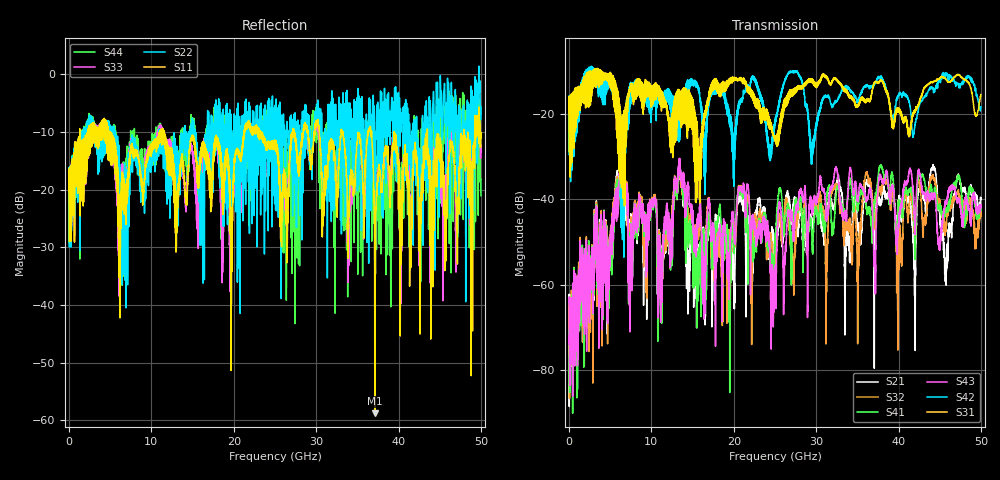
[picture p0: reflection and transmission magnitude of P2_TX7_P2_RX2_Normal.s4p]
!Keysight Technologies,N5225B,MY57041031,A.13.20.10
!Date: Friday, May 31, 2019 11:29:40
!Correction: S11(Full 4 Port(1,2,3,4))
!S12(Full 4 Port(1,2,3,4))
!S13(Full 4 Port(1,2,3,4))
!S14(Full 4 Port(1,2,3,4))
!S21(Full 4 Port(1,2,3,4))
!S22(Full 4 Port(1,2,3,4))
!S23(Full 4 Port(1,2,3,4))
!S24(Full 4 Port(1,2,3,4))
!S31(Full 4 Port(1,2,3,4))
!S32(Full 4 Port(1,2,3,4))
!S33(Full 4 Port(1,2,3,4))
!S34(Full 4 Port(1,2,3,4))
!S41(Full 4 Port(1,2,3,4))
!S42(Full 4 Port(1,2,3,4))
!S43(Full 4 Port(1,2,3,4))
!S44(Full 4 Port(1,2,3,4))
!S4P File: Measurements: <S11,S12,S13,S14>,
!<S21,S22,S23,S24>,
!<S31,S32,S33,S34>,
!<S41,S42,S43,S44>:
# Hz S  dB  R 50.0
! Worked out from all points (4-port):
!   5000 points, 10 MHz to 50 GHz, reference 50 ohm
!   strongest paths, dB at 10 MHz, 12.51 GHz, 25.01 GHz, 37.51 GHz, 50 GHz:
!     S31: -19.7, -21.3, -25.9, -12.8, -15.4
!     S42: -19.3, -16.0, -21.7, -11.4, -18.3
!     S43: -62.9, -52.0, -56.0, -37.4, -41.5
!     S41: -70.6, -53.9, -49.7, -34.9, -41.9
!     S32: -65.4, -46.4, -53.9, -37.9, -43.0
!     S21: -64.2, -46.6, -55.9, -38.4, -39.6
!   lowest |S11| = -58.8 dB at 37.12 GHz (marker M1), VSWR 1.00, Z = 49.9 - j0.0234 ohm
!   |S11| at or under -10 dB: 4.911 GHz to 11.03 GHz (6.116 GHz wide, 76.7 % of centre); 11.57 GHz to 21.26 GHz (9.684 GHz wide, 59 % of centre); 43.5 GHz to 47.91 GHz (4.407 GHz wide, 9.64 % of centre)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
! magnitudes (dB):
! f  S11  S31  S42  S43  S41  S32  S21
! 10 MHz  -20.2  -19.7  -19.3  -62.9  -70.6  -65.4  -64.2
! 6.36 GHz  -18.7  -25.4  -32.1  -34.5  -37.2  -37.4  -41.7
! 11.02 GHz  -10.6  -17.6  -16.9  -54.9  -54.0  -52.2  -52.8
! 13.43 GHz  -18.4  -21.1  -26.1  -30.4  -31.5  -30.6  -31.7
! 15.36 GHz  -12.8  -40.7  -13.1  -48.4  -51.5  -48.5  -52.4
! 37.12 GHz  -58.8  -12.6  -12.8  -58.1  -40.7  -46.9  -49.4
! 50 GHz  -11.1  -15.4  -18.3  -41.5  -41.9  -43.0  -39.6
